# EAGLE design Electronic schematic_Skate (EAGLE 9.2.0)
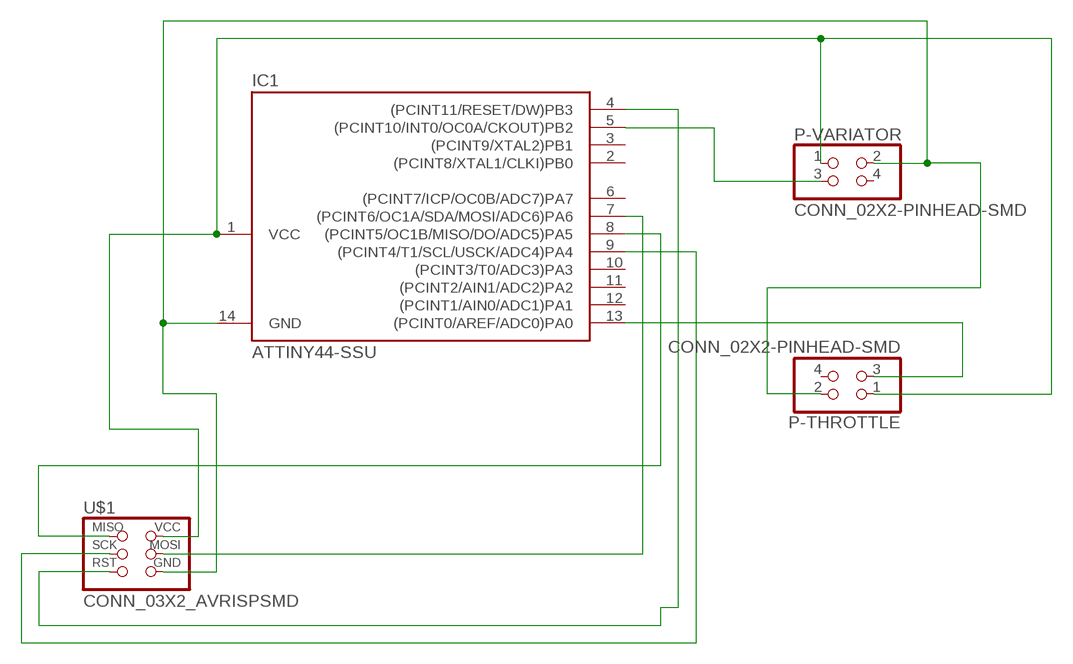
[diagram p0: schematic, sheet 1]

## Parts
IC1  ATTINY44-SSU  [SOIC14]
P-THROTTLE  CONN_02X2-PINHEAD-SMD  [2X02SMD]
P-VARIATOR  CONN_02X2-PINHEAD-SMD  [2X02SMD]
U$1  CONN_03X2_AVRISPSMD  [2X03SMD]

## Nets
N$1: IC1.1(VCC) P-THROTTLE.1 P-VARIATOR.1 U$1.2(VCC)
N$2: IC1.14(GND) P-THROTTLE.2 P-VARIATOR.2 U$1.6(GND)
N$3: IC1.4((PCINT11/RESET/DW)PB3) U$1.5(RST)
N$4: IC1.9((PCINT4/T1/SCL/USCK/ADC4)PA4) U$1.3(SCK)
N$5: IC1.7((PCINT6/OC1A/SDA/MOSI/ADC6)PA6) U$1.4(MOSI)
N$6: IC1.8((PCINT5/OC1B/MISO/DO/ADC5)PA5) U$1.1(MISO)
N$7: IC1.5((PCINT10/INT0/OC0A/CKOUT)PB2) P-VARIATOR.3
N$10: IC1.13((PCINT0/AREF/ADC0)PA0) P-THROTTLE.3
Unconnected: IC1.2((PCINT8/XTAL1/CLKI)PB0) IC1.3((PCINT9/XTAL2)PB1) IC1.6((PCINT7/ICP/OC0B/ADC7)PA7) IC1.10((PCINT3/T0/ADC3)PA3) IC1.11((PCINT2/AIN1/ADC2)PA2) IC1.12((PCINT1/AIN0/ADC1)PA1) P-THROTTLE.4 P-VARIATOR.4

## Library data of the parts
IC1 = fab:ATTINY44
P-THROTTLE P-VARIATOR = fab:CONN_02X2-PINHEAD-SMD
U$1 = fab:CONN_03X2_AVRISP

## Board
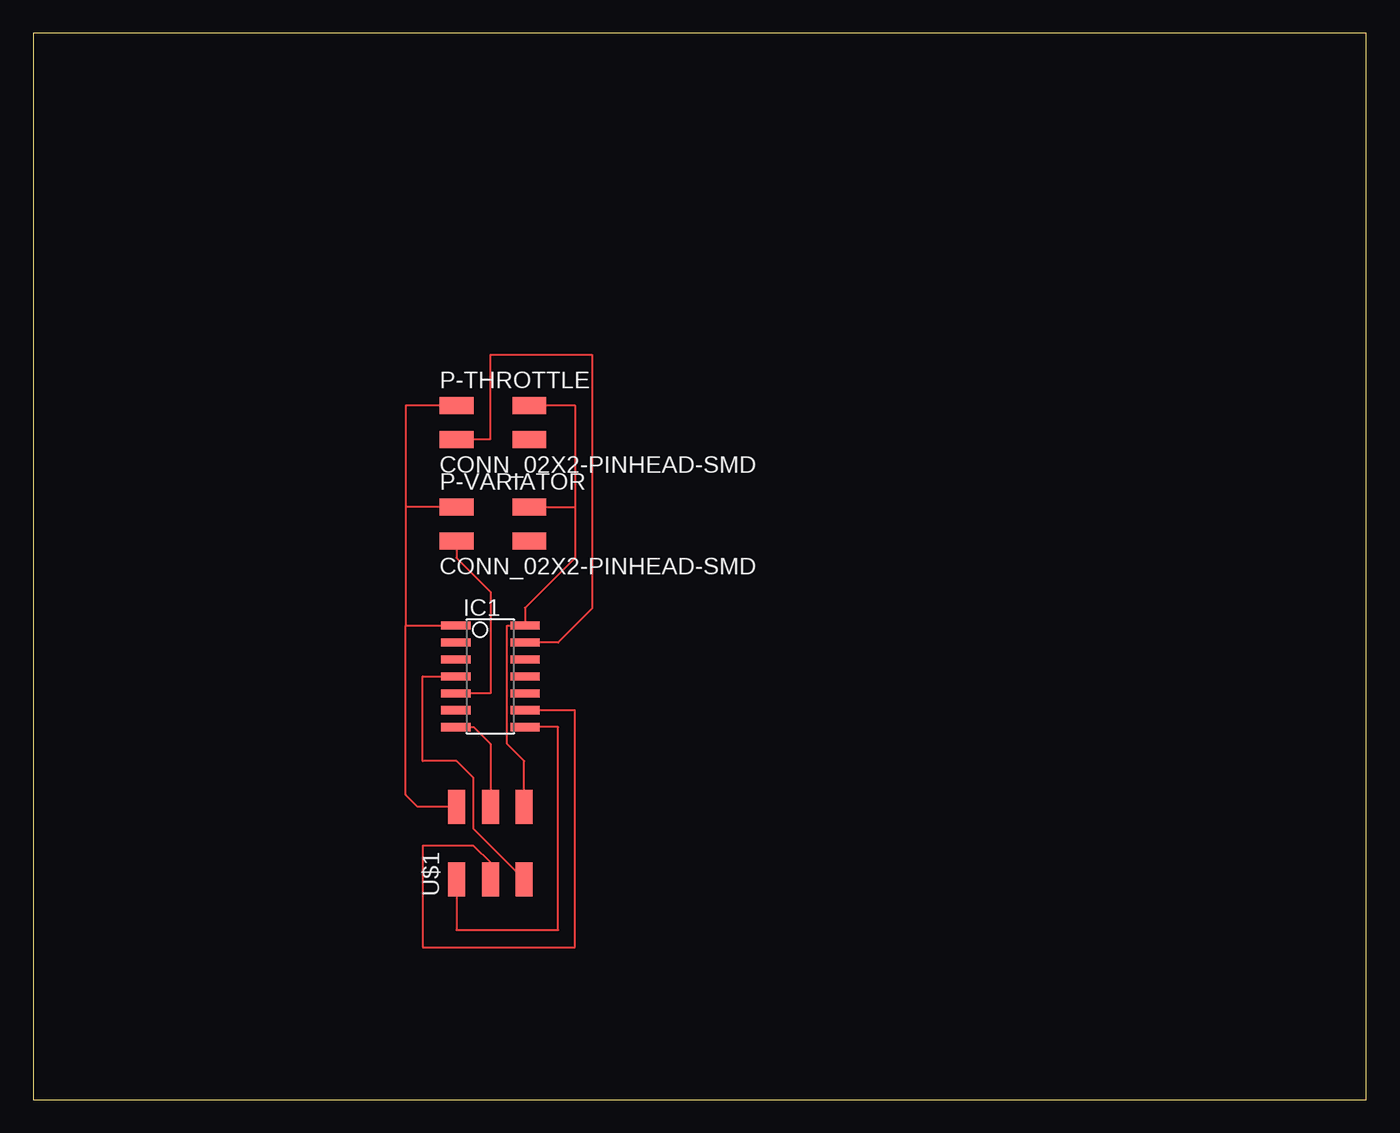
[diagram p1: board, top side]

Size 100 x 80 mm. Coordinates in mm from the lower left corner, seen from the top.
Outline: 0,0 100,0 100,80 0,80 0,0
Copper layers (1*16): Top 0.035mm / dielectric 1.5mm / Bottom 0.035mm
Design rules "default": minimum track width 6mil, minimum drill 0.35mm, track to track 6mil, track to pad 6mil, pad to pad 6mil, via to via 6mil, smd to smd 6mil, copper to edge 40mil, drill to drill 6mil, minimum pad ring 10mil, minimum via ring 8mil, stop-mask expansion 4mil, vias tented up to drill 0mil, thermal gap 10mil

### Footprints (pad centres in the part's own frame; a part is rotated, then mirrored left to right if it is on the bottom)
SOIC14 = smd 0.61 x 2.21: 1 -3.81,-2.603; 2 -2.54,-2.603; 3 -1.27,-2.603; 4 0,-2.603; 5 1.27,-2.603; 6 2.54,-2.603; 7 3.81,-2.603; 8 3.81,2.603; 9 2.54,2.603; 10 1.27,2.603; 11 0,2.603; 12 -1.27,2.603; 13 -2.54,2.603; 14 -3.81,2.603
2X02SMD = smd 2.54 x 1.27: 1 -2.54,1.27; 2 2.92,1.27; 3 -2.54,-1.27; 4 2.92,-1.27
2X03SMD = smd 2.54 x 1.27: 1 -2.54,2.54; 2 2.92,2.54; 3 -2.54,0; 4 2.92,0; 5 -2.54,-2.54; 6 2.92,-2.54

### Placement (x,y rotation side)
IC1  34.29,31.75 270 top
P-THROTTLE  34.29,50.8 0 top
P-VARIATOR  34.29,43.18 0 top
U$1  34.29,19.05 90 top

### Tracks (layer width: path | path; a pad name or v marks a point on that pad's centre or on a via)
N$1
  Top 0.152: U$1.2 28.83,21.97 27.94,22.86 27.94,35.56 | 27.94,35.56 IC1.1 | P-VARIATOR.1 27.94,44.45 | 27.94,44.45 27.94,35.56 | P-THROTTLE.1 27.94,52.07 27.94,44.45
N$2
  Top 0.152: P-VARIATOR.2 40.64,44.45 | 40.64,44.45 40.64,40.64 36.89,36.89 IC1.14 35.56,35.56 35.56,26.67 36.83,25.4 U$1.6 | P-THROTTLE.2 40.64,52.07 40.64,44.45
N$3
  Top 0.152: U$1.5 33.02,20.32 33.02,24.13 31.75,25.4 29.21,25.4 29.21,31.75 IC1.4
N$4
  Top 0.152: U$1.3 34.29,17.78 33.02,19.05 29.21,19.05 29.21,11.43 40.64,11.43 40.64,29.21 IC1.9
N$5
  Top 0.152: U$1.4 34.29,26.67 33.02,27.94 IC1.7
N$6
  Top 0.152: U$1.1 31.75,12.7 39.37,12.7 39.37,27.94 IC1.8
N$7
  Top 0.152: P-VARIATOR.3 31.75,40.64 34.29,38.1 34.29,30.48 IC1.5
N$10
  Top 0.152: P-THROTTLE.3 34.29,49.53 34.29,55.88 41.91,55.88 41.91,36.83 39.37,34.29 IC1.13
